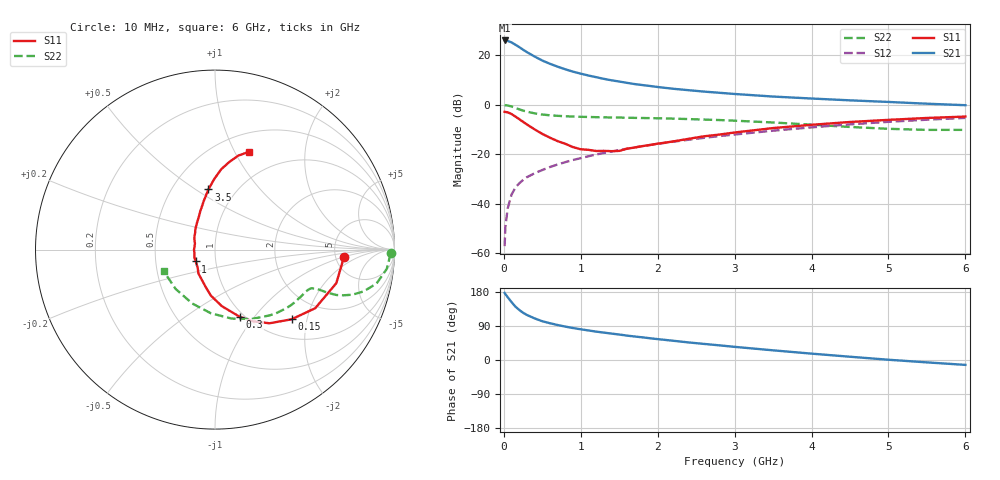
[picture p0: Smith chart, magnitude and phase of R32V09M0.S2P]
! SIEMENS Small Signal Semiconductors
! BFR181
! Si NPN RF Bipolar Junction Transistor in SOT23
! VCE = 2 V  IC = 9 mA
! Common Emitter S-Parameters:  May  1996
# GHz  S  MA  R  50
!  f  S11  S21  S12  S22
! GHz  MAG  ANG  MAG  ANG  MAG  ANG  MAG  ANG
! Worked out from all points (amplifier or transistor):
!   36 points, 10 MHz to 6 GHz, reference 50 ohm
!   highest |S21| = 25.9 dB at 10 MHz (marker M1)
!   |S21| within 3 dB of that: start of sweep to 215.6 MHz
!   unconditionally stable (mu >= 1): 725.6 MHz to 2.694 GHz
!   at 250 MHz: K = 0.61, MSG = 26.3 dB, |S12| = -30.4 dB
!   at 1.4 GHz: K = 1.09, MAG = 12.6 dB, |S12| = -18.9 dB
!   at 6 GHz: K = 0.86, MSG = 2.6 dB, |S12| = -5.3 dB
!   S11 on the Smith chart (normalised r, x): 10 MHz: 5.91, -1.04; 150 MHz: 1.39, -1.62; 300 MHz: 0.95, -0.85; 1 GHz: 0.80, -0.11; 3.5 GHz: 0.75, +0.57; 6 GHz: 0.70, +1.14
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0.01  0.7182 -3.4  19.73 177.0  0.0014 90.8  0.9791 -1.2
0.02  0.7122 -6.3  19.41 174.0  0.0034 86.6  0.9741 -2.6
0.05  0.7012 -15.5  19.33 165.7  0.0081 83.0  0.9631 -6.4
0.1  0.647 -30.3  17.98 152.8  0.0153 77.5  0.9195 -11.9
0.15  0.5769 -42.3  16.19 141.0  0.0213 71.7  0.8602 -15.7
0.2  0.5107 -53.5  14.5 132.1  0.0259 69.3  0.8054 -18.2
0.25  0.4507 -62.3  12.86 124.7  0.0303 66.9  0.7587 -19.6
0.3  0.399 -69.8  11.47 118.8  0.0345 67.3  0.7226 -20.5
0.4  0.3173 -83.1  9.355 109.8  0.0414 66.2  0.6687 -21.0
0.5  0.2572 -95.2  7.76 102.3  0.0481 67.0  0.6328 -21.0
0.6  0.2156 -103.8  6.674 97.0  0.0553 67.5  0.6104 -21.1
0.7  0.1838 -113.5  5.838 92.3  0.0623 68.3  0.5956 -21.3
0.8  0.1621 -124.7  5.16 88.1  0.0694 68.3  0.5842 -21.7
1  0.126 -148.3  4.219 81.0  0.0836 69.1  0.5697 -22.7
1.1  0.1228 -159.5  3.874 78.0  0.0911 69.2  0.5645 -23.5
1.3  0.1171 -179.3  3.318 72.3  0.1061 69.1  0.5554 -25.3
1.6  0.1293 153.1  2.756 64.4  0.1295 68.3  0.5456 -28.6
2.2  0.1812 123.4  2.094 50.8  0.179 65.6  0.5227 -36.8
3.5  0.3374 96.2  1.458 25.5  0.2986 55.1  0.4373 -62.1
4.5  0.4478 85.7  1.223 8.6  0.4006 43.8  0.3554 -93.7
5.5  0.5394 76.1  1.046 -6.3  0.4978 30.4  0.3101 -135.1
6  0.5753 71.0  0.976 -12.9  0.541 23.0  0.3104 -157.5
